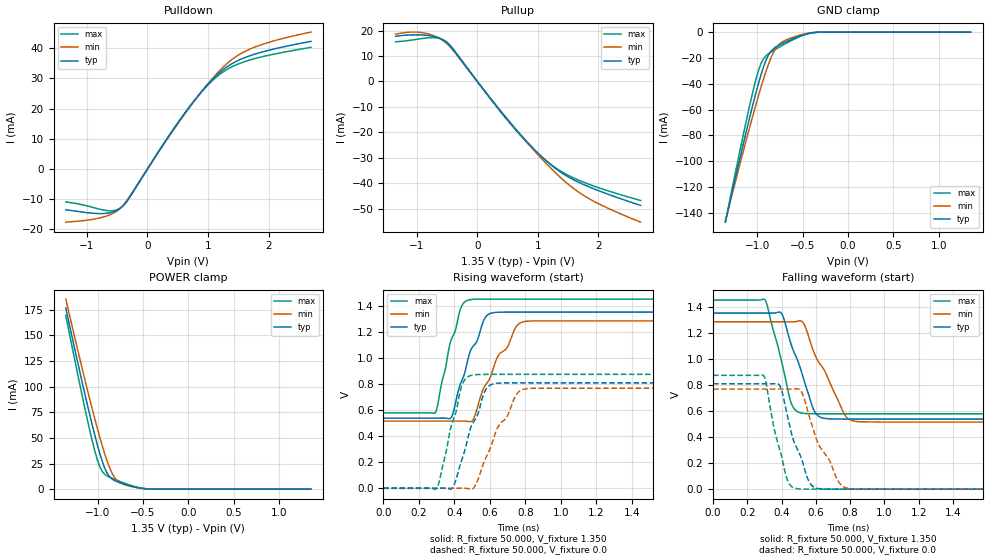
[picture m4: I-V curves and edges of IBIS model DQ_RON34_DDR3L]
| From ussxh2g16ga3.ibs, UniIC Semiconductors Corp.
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|   Model DQ_RON34_DDR3L
[Model] DQ_RON34_DDR3L
Model_type I/O
Vinl =  0.540V
Vinh =  0.810V
Vmeas =  0.675V
Rref =  50.000
Vref =  0.675V
C_comp   0.966pF   0.965pF   0.967pF
[Model Spec]
Vinh   0.810V   0.776V   0.860V
Vinl   0.540V   0.506V   0.590V
Vmeas   0.675V   0.641V   0.725V
Vref   0.675V   0.641V   0.725V
Rref   50.000   NA   NA
[Temperature Range]   25.000   95.000   -40.000
[Voltage Range]   1.350V   1.283V   1.450V
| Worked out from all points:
|   slope of the pulldown table from 0 to 0.203 V, typ, clamps not added: 31.9 ohm
|   slope of the pullup table from 0 to 0.203 V, typ, clamps not added: 32.6 ohm
|   GND clamp passes 1 mA (typ) near -0.43 V on its own axis
|   POWER clamp passes 1 mA (typ) near -0.52 V on its own axis
|   rising waveform, R_fixture 50.000, V_fixture 1.350: 20-80 % time 128ps typ, 174ps min, 95.7ps max; typ from 0.537 V to 1.35 V
|   rising waveform, R_fixture 50.000, V_fixture 0.0: 20-80 % time 120ps typ, 161ps min, 90.6ps max; typ from 0 V to 0.808 V
|   falling waveform, R_fixture 50.000, V_fixture 1.350: 20-80 % time 125ps typ, 167ps min, 97.4ps max; typ from 1.35 V to 0.537 V
|   falling waveform, R_fixture 50.000, V_fixture 0.0: 20-80 % time 113ps typ, 150ps min, 88.6ps max; typ from 0.808 V to 0 V
[Pulldown]
|Voltage   I(typ)   I(min)   I(max)
-1.35V    -13.51mA   -17.62mA   -10.91mA
-735mV    -14.75mA   -15.95mA   -13.56mA
-571mV    -14.25mA   -14.71mA   -13.81mA
-448mV    -12.99mA   -12.97mA   -12.94mA
-325mV    -10.21mA   -9.97mA    -10.3mA
249mV     7.763mA    7.591mA    7.831mA
618mV     18.51mA    18.29mA    18.54mA
905mV     25.92mA    25.92mA    25.74mA
1.151V    31.18mA    31.69mA    30.65mA
1.397V    34.88mA    36.26mA    33.86mA
1.684V    37.44mA    39.62mA    36.03mA
2.7V      42.25mA    45.33mA    40.28mA
[Pullup]
|Voltage   I(typ)   I(min)   I(max)
-1.35V    17.72mA    18.59mA    15.57mA
-908mV    18.24mA    19.13mA    16.88mA
-703mV    17.58mA    17.82mA    17.17mA
-539mV    15.84mA    15.58mA    16.08mA
-416mV    12.97mA    12.65mA    13.32mA
568mV     -16.88mA   -16.85mA   -17.2mA
855mV     -24.54mA   -24.84mA   -24.81mA
1.142V    -31.21mA   -32.28mA   -31.21mA
1.429V    -36.41mA   -38.87mA   -35.92mA
1.757V    -40.49mA   -44.75mA   -39.57mA
2.126V    -43.98mA   -49.41mA   -42.68mA
2.7V      -48.67mA   -55.27mA   -46.75mA
[GND_clamp]
|Voltage   I(typ)   I(min)   I(max)
-1.35V    -146.9mA   -146.3mA   -147.1mA
-1.126V   -78.8mA    -85.17mA   -70.77mA
-1.014V   -47.25mA   -56.31mA   -36.92mA
-958mV    -33.17mA   -42.77mA   -24.44mA
-930mV    -26.97mA   -36.36mA   -20.61mA
-874mV    -17.51mA   -24.69mA   -16.72mA
-818mV    -12.71mA   -15.46mA   -14.21mA
-762mV    -10.26mA   -9.751mA   -11.88mA
-706mV    -8.307mA   -6.907mA   -9.644mA
-538mV    -3.274mA   -2.499mA   -3.731mA
-398mV    -591.2uA   -439.3uA   -663.7uA
1.35V     0A         0A         0A
[POWER_clamp]
|Voltage   I(typ)   I(min)   I(max)
-1.35V    176.6mA    185.4mA    169.4mA
-1.198V   115.5mA    128.2mA    103.2mA
-1.114V   83.04mA    97.6mA     68.48mA
-1.058V   62.42mA    77.92mA    46.98mA
-1.002V   43.19mA    59.09mA    28.56mA
-946mV    26.54mA    41.57mA    16.92mA
-890mV    14.85mA    26.22mA    12.66mA
-834mV    9.439mA    14.55mA    10.39mA
-778mV    7.089mA    7.901mA    8.361mA
-638mV    3.198mA    2.764mA    3.815mA
-414mV    126.6uA    165.9uA    94.28uA
1.35V     0A         0A         0A
[Ramp]
| variable   typ   min   max
dV/dt_r   0.485/0.120n   0.460/0.161n   0.524/90.705p
dV/dt_f   0.488/0.125n   0.461/0.167n   0.523/97.430p
R_load = 50.000
[Rising Waveform]
R_fixture= 50.000
V_fixture= 1.350
V_fixture_min= 1.283
V_fixture_max= 1.450
|time   V(typ)   V(min)   V(max)
0s        537.3mV    514.5mV    578mV
293ps     537.3mV    514.5mV    580mV
383ps     543.8mV    514.5mV    1.141V
441ps     822.3mV    515mV      1.396V
484ps     1.028V     510.4mV    1.444V
513ps     1.1V       546.3mV    1.449V
586ps     1.327V     810.8mV    1.45V
651ps     1.349V     1.025V     1.45V
788ps     1.35V      1.276V     1.45V
3ns       1.35V      1.283V     1.45V
[Rising Waveform]
R_fixture= 50.000
V_fixture= 0.0
V_fixture_min= 0.0
V_fixture_max= 0.0
|time   V(typ)   V(min)   V(max)
0s        140.3nV    915.5nV    76.88nV
299ps     -79.46uV   2.931uV    -2.765mV
397ps     20.76mV    -61.67uV   535mV
445ps     229.9mV    555.2uV    797.7mV
496ps     478.8mV    -6.818mV   865.7mV
586ps     773.7mV    257mV      872.7mV
641ps     804.9mV    459.5mV    872.8mV
747ps     807.9mV    714.6mV    872.9mV
789ps     807.9mV    758.4mV    872.9mV
3ns       807.9mV    767.3mV    872.9mV
[Falling Waveform]
R_fixture= 50.000
V_fixture= 1.350
V_fixture_min= 1.283
V_fixture_max= 1.450
|time   V(typ)   V(min)   V(max)
0s        1.35V      1.283V     1.45V
301ps     1.35V      1.283V     1.455V
400ps     1.347V     1.283V     977.1mV
457ps     1.104V     1.283V     656.3mV
511ps     920.5mV    1.291V     584.9mV
577ps     642.9mV    1.09V      578.3mV
613ps     562.1mV    980.2mV    578mV
764ps     537.4mV    579.1mV    578mV
827ps     537.3mV    520.4mV    578mV
3ns       537.3mV    514.5mV    578mV
[Falling Waveform]
R_fixture= 50.000
V_fixture= 0.0
V_fixture_min= 0.0
V_fixture_max= 0.0
|time   V(typ)   V(min)   V(max)
0s        807.9mV    767.3mV    872.9mV
293ps     807.9mV    767.3mV    873mV
390ps     792.3mV    767.3mV    298.3mV
435ps     555.7mV    767.1mV    65.69mV
483ps     331.2mV    769mV      5.593mV
521ps     214.2mV    733.2mV    782.1uV
584ps     19.73mV    462.8mV    31.59uV
722ps     36.48uV    81.4mV     250.5nV
783ps     2.599uV    7.159mV    201.6nV
3ns       78.32nV    867.5nV    130.3nV
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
